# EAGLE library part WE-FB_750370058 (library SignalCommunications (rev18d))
WE-FB Flyback Transformer suitable for LT3573/ LT3574/ LT3575/ LT3748 Characteristics easy design in solution less external components needed small board space low cost no optocoupler needed! long term reliability voltage control no aging same external parts for different output voltages easy design of custom power supply due to standard circuit and change of transformers and two components for feedback loop Isolation voltage up to 2.5 kV Applications Isolated power design Sensor interfaces Isolated telecom converters Power over Ethernet Details see: http://katalog.we-online.de/en/pbs/WE-FB_Linear? Updated 2014-07-07 2014 (C) Wurth Elektronik
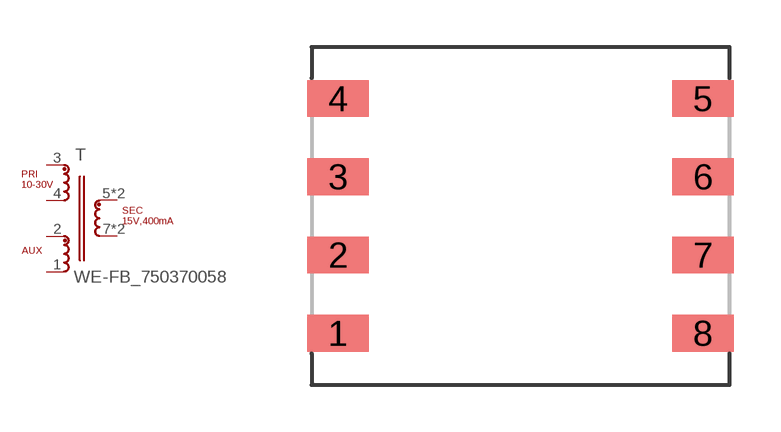
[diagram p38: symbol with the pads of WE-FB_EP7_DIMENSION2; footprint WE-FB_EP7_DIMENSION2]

Designator prefix T

## WE-FB_750370058  [WE-FB_EP7_DIMENSION2]
1  4  pas
2  5  pas
3  1  pas
4  6  pas
5  2  pas
6  2  pas
7  3  pas
8  3  pas

## Footprint WE-FB_EP7_DIMENSION2 (pad centres in mm)
Transformer, EP7* SMD 8Pin für WE-FB
smd 1.96 x 1.17: 1 -5.83,-3.75; 2 -5.83,-1.25; 3 -5.83,1.25; 4 -5.83,3.75; 5 5.83,3.75; 6 5.83,1.25; 7 5.83,-1.25; 8 5.83,-3.75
